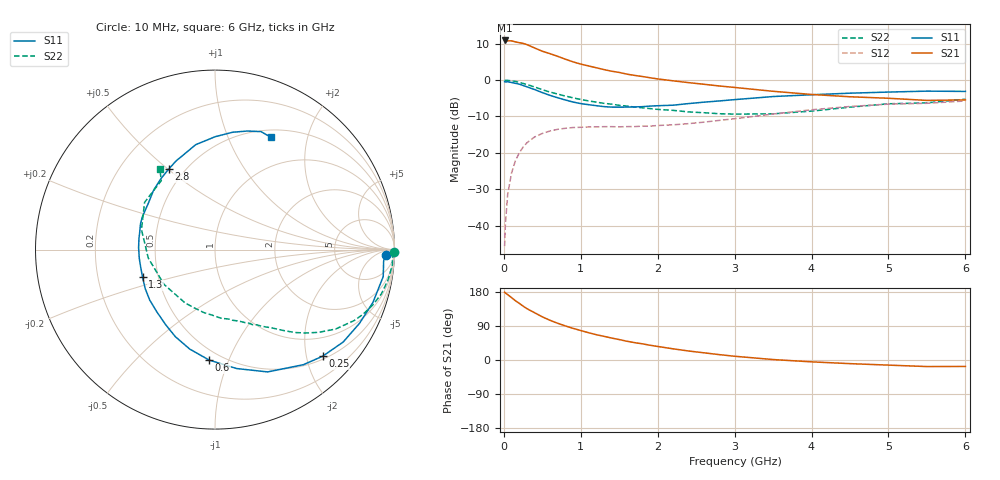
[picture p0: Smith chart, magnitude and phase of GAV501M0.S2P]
! Infineon Technologies  Discrete & RF Semiconductors
! BF775
! Si NPN RF Bipolar Junction Transistor in SOT23
! VCE = 0.5 V  IC = 1 mA
! Common Emitter S-Parameters:  May  1996
# GHz  S  MA  R  50
!  f  S11  S21  S12  S22
! GHz  MAG  ANG  MAG  ANG  MAG  ANG  MAG  ANG
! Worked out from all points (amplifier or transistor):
!   36 points, 10 MHz to 6 GHz, reference 50 ohm
!   highest |S21| = 10.9 dB at 10 MHz (marker M1)
!   |S21| within 3 dB of that: start of sweep to 505.1 MHz
!   unconditionally stable (mu >= 1): 1.264 GHz to end of sweep
!   at 250 MHz: K = 0.23, MSG = 14.3 dB, |S12| = -18.4 dB
!   at 1.4 GHz: K = 1.08, MAG = 5.9 dB, |S12| = -12.8 dB
!   at 6 GHz: K = 1.12, MAG = -2.0 dB, |S12| = -5.7 dB
!   S11 on the Smith chart (normalised r, x): 10 MHz: 28, -19; 250 MHz: 0.56, -2.32; 600 MHz: 0.43, -0.85; 1.3 GHz: 0.41, -0.15; 2.8 GHz: 0.41, +0.50; 6 GHz: 0.59, +1.44
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0.01  0.9517 -1.9  3.512 178.8  0.0052 89.3  0.9974 -0.9
0.02  0.9417 -3.8  3.459 176.8  0.0103 88.1  0.9896 -2.0
0.05  0.9492 -9.1  3.466 172.4  0.0269 84.1  0.9918 -5.1
0.1  0.9279 -18.5  3.466 164.7  0.0526 78.2  0.978 -10.1
0.15  0.9037 -27.1  3.36 156.5  0.0776 72.4  0.9594 -14.9
0.25  0.8443 -44.7  3.204 142.2  0.1198 61.7  0.9002 -23.6
0.3  0.8084 -52.5  3.078 135.5  0.1375 57.7  0.8705 -27.0
0.4  0.742 -66.7  2.769 124.7  0.1652 49.6  0.8043 -33.4
0.5  0.6735 -79.7  2.496 113.9  0.1847 43.0  0.7388 -38.6
0.6  0.6165 -93.0  2.311 104.8  0.1996 37.7  0.6854 -42.7
0.7  0.572 -104.2  2.124 96.9  0.2106 33.5  0.6434 -45.9
0.8  0.533 -114.5  1.94 89.9  0.2175 30.0  0.6034 -48.8
0.9  0.4993 -123.7  1.783 83.5  0.2228 27.4  0.5708 -51.3
1.1  0.4597 -142.4  1.568 72.1  0.2268 23.5  0.5179 -56.4
1.3  0.4321 -159.1  1.397 62.5  0.2289 21.0  0.4797 -60.9
1.7  0.4281 171.8  1.161 45.8  0.2295 20.1  0.4258 -70.3
2.2  0.452 145.4  0.978 29.5  0.2427 22.5  0.384 -84.9
2.8  0.517 120.0  0.831 14.2  0.2793 25.2  0.345 -109.2
3.5  0.5944 100.4  0.702 1.2  0.3415 23.1  0.3438 -145.6
4.5  0.6614 81.4  0.59 -9.6  0.434 13.3  0.4245 164.8
5.5  0.7055 68.7  0.526 -17.3  0.4799 -0.2  0.4869 127.9
6  0.6991 63.6  0.535 -17.0  0.5168 -3.8  0.5462 124.3
